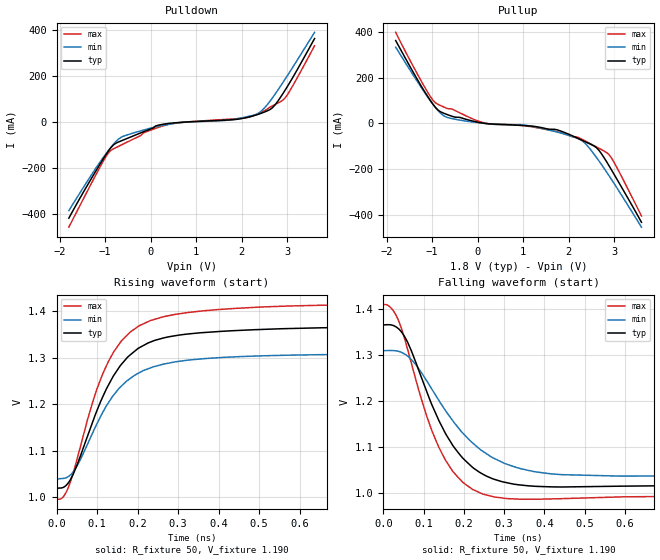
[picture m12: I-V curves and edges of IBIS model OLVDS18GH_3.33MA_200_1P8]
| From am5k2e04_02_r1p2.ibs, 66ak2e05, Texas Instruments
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|   Model Cell OLVDS18GH_3.33MA_200_1P8
|olvds18gh.ibs [30Dec11 revision 1.0]
|OLVDS18GH_3.33MA_200_1P8
[Model]   OLVDS18GH_3.33MA_200_1P8
Model_type   Output
Polarity   Non-Inverting
Cref =  15.0001pF
Rref =  101.0000M
Vref =  0V
Vmeas =  1.08V
C_comp   1p   1p   1p
[Temperature Range]   25   125   -40
[Voltage Range]   1.8   1.62   1.98
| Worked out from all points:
|   slope of the pulldown table from 0 to 0.27 V, typ, clamps not added: 13.4 ohm
|   slope of the pullup table from 0 to 0.27 V, typ, clamps not added: 36.4 ohm
|   rising waveform, R_fixture 50, V_fixture 1.190: 20-80 % time 111ps typ, 116ps min, 103ps max; typ from 1.02 V to 1.36 V
|   falling waveform, R_fixture 50, V_fixture 1.190: 20-80 % time 109ps typ, 142ps min, 93.8ps max; typ from 1.36 V to 1.02 V
| Nom Voltages:
[Pulldown]
|   voltage   I(typ)   I(min)   I(max)
-1.8V     -417.4mA   -384.6mA   -456.3mA
-1.091V   -174.6mA   -166.6mA   -186.2mA
-872.7mV  -110mA     -108.6mA   -121.9mA
-600mV    -77.11mA   -60.8mA    -94.41mA
163.6mV   -13.13mA   -17.75mA   -22.77mA
545.5mV   -2.35mA    -4.57mA    -3.714mA
1.691V    9.579mA    9.125mA    12.96mA
2.073V    18.77mA    22.25mA    19.16mA
2.345V    33.34mA    36.94mA    35.73mA
2.673V    62.83mA    105.5mA    71.06mA
2.945V    137.3mA    185.3mA    104.1mA
3.6V      364.1mA    391mA      333.1mA
[Pullup]
|   voltage   I(typ)   I(min)   I(max)
-1.8V     360.9mA    332.1mA    396.7mA
-1.145V   132.7mA    129.3mA    152.2mA
-981.8mV  84.17mA    83.58mA    101.1mA
-872.7mV  58.8mA     56.74mA    83.51mA
-654.5mV  37.83mA    25.7mA     64.21mA
163.6mV   184.2uA    311uA      1.888mA
981.8mV   -8.727mA   -5.823mA   -9.071mA
1.691V    -25.33mA   -34.52mA   -33.39mA
2.291V    -72.63mA   -74.49mA   -68.68mA
2.618V    -106.6mA   -149.9mA   -102.8mA
2.891V    -185.2mA   -228.3mA   -136.3mA
3.6V      -430.1mA   -451.3mA   -402.8mA
[Ramp]
| variable   typ   min   max
dV/dt_f   11.172m/1.2939n   3.84m/0.90862922n   5.406m/0.64911174n
dV/dt_r   5.562m/1.1684491n   3.738m/3.4802345n   4.788m/0.60624971n
R_load = 50
[Rising Waveform]
R_fixture = 50
V_fixture = 1.190
V_fixture_min = 1.1743
V_fixture_max = 1.20176
|   time   V(typ)   V(min)   V(max)
0s        1.019V     1.039V     995.6mV
21.2ps    1.023V     1.041V     1.006V
40.3ps    1.048V     1.054V     1.049V
97.3ps    1.181V     1.153V     1.226V
140.1ps   1.26V      1.218V     1.311V
200ps     1.319V     1.265V     1.366V
256.6ps   1.341V     1.284V     1.386V
402.3ps   1.356V     1.3V       1.403V
689.7ps   1.365V     1.307V     1.413V
1.724ns   1.365V     1.309V     1.41V
[Falling Waveform]
R_fixture = 50
V_fixture = 1.190
V_fixture_min = 1.1743
V_fixture_max = 1.20176
|   time   V(typ)   V(min)   V(max)
0s        1.365V     1.309V     1.409V
25.5ps    1.363V     1.309V     1.395V
52.7ps    1.339V     1.302V     1.335V
108.2ps   1.218V     1.242V     1.165V
151.9ps   1.132V     1.181V     1.074V
194.8ps   1.077V     1.131V     1.024V
246ps     1.04V      1.09V      996.9mV
335.7ps   1.017V     1.053V     985.4mV
442.2ps   1.012V     1.039V     986.6mV
1.262ns   1.019V     1.039V     995.5mV
